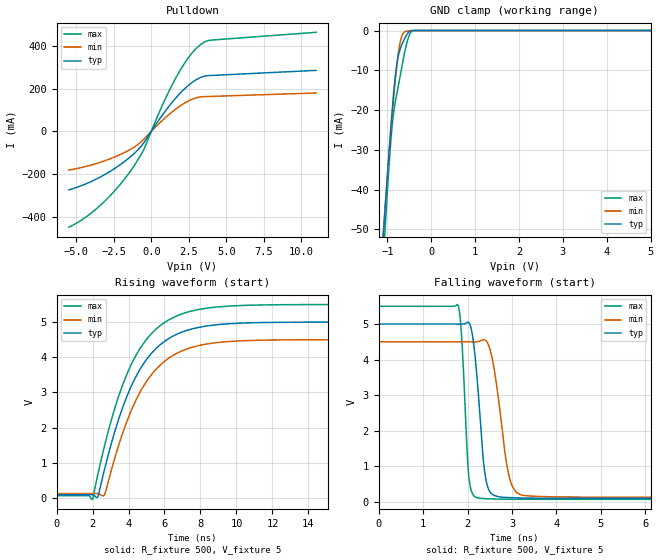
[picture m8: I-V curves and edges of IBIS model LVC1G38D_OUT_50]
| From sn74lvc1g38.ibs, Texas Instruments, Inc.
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[Model]   LVC1G38D_OUT_50
Model_type  Open_drain
Enable   Active-High
Vref =   5.0
Rref =   500
Cref =   50p
Vmeas =   2.5
| variable   typ   min   max
C_comp   3.59pF   2.67pF   5.07pF
| C_pulldown   6.34pF   4.47pF   9.75pF
| C_tri-state   3.59pF   2.67pF   5.07pF
[Temperature Range]   40   100   -40
| Ambient temperature   25   85   -40
[Voltage range]   5   4.5   5.5
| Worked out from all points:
|   slope of the pulldown table from 0 to 0.75 V, typ, clamps not added: 9.74 ohm
|   GND clamp passes 1 mA (typ) near -0.56 V on its own axis
|   rising waveform, R_fixture 500, V_fixture 5: 20-80 % time 2.33ns typ, 2.31ns min, 2.35ns max; typ from 0.091 V to 5 V
|   falling waveform, R_fixture 500, V_fixture 5: 20-80 % time 188ps typ, 277ps min, 125ps max; typ from 5 V to 0.091 V
[GND Clamp]
| LVC1G38D_OUT_50
|   Voltage   I(typ)   I(min)   I(max)
-5.5V     -916.4mA   -845.5mA   -1.045A
-1.09V    -50.76mA   -49.98mA   -56.67mA
-1.06V    -45.77mA   -45.39mA   -51.02mA
-1.045V   -43.3mA    -43.11mA   -48.24mA
-915mV    -23.14mA   -24.32mA   -26.62mA
-870mV    -17.04mA   -18.38mA   -21.54mA
-820mV    -11.32mA   -12.35mA   -17.86mA
-765mV    -7.029mA   -6.772mA   -14.61mA
-710mV    -4.653mA   -2.903mA   -11.41mA
-590mV    -1.618mA   -231.3uA   -4.549mA
-430mV    -5.996uA   -38.1uA    -30.86uA
5V        30.43pA    275.2pA    975.5pA
[Pulldown]
| LVC1G38D_OUT_50
|   Voltage   I(typ)   I(min)   I(max)
-5.5V     -273.4mA   -180.8mA   -448mA
-4.485V   -248.9mA   -166.3mA   -406.7mA
-3.435V   -214.6mA   -145.3mA   -347.9mA
-2.39V    -171.2mA   -118.1mA   -273.7mA
-1.44V    -121.8mA   -85.93mA   -190.7mA
-515mV    -55.2mA    -37.6mA    -87.68mA
715mV     73.64mA    49.68mA    118.1mA
1.685V    159.9mA    107mA      255.9mA
2.51V     217.1mA    143.2mA    347.6mA
3.26V     251.1mA    161mA      404.3mA
3.945V    261.2mA    163.3mA    426.7mA
11V       285.2mA    179.5mA    463.2mA
[Ramp]
| LVC1G38D_OUT_50
| variable   typ   min   max
dV/dt_r   2.99/2.33E-09   2.67/2.32E-09   3.33/2.35E-09
dV/dt_f   2.98/1.95E-10   2.66/2.90E-10   3.29/1.28E-10
R_load = 500
[Rising Waveform]
| LVC1G38D_OUT_50
R_fixture =   500
C_fixture =   0
L_fixture =   0
V_fixture =   5
V_fixture_min = 4.5
V_fixture_max = 5.5
|   Time   V(typ)   V(min)   V(max)
0s        91.33mV    120.7mV    62.82mV
2.01ns    91.31mV    120.7mV    -34.92mV
2.305ns   40.65mV    120.7mV    683.9mV
2.665ns   805.5mV    88.22mV    1.471V
3.365ns   2.097V     1.351V     2.755V
4.07ns    3.082V     2.382V     3.704V
5.245ns   4.093V     3.484V     4.655V
6.69ns    4.656V     4.113V     5.178V
10.38ns   4.973V     4.47V      5.474V
24.99ns   5V         4.5V       5.5V
[Falling Waveform]
| LVC1G38D_OUT_50
R_fixture =   500
C_fixture =   0
L_fixture =   0
V_fixture =   5
V_fixture_min = 4.5
V_fixture_max = 5.5
|   Time   V(typ)   V(min)   V(max)
0s        5V         4.5V       5.5V
1.785ns   4.999V     4.5V       5.527V
1.87ns    4.998V     4.5V       4.557V
2.03ns    5.039V     4.499V     683.9mV
2.255ns   2.83V      4.512V     97.86mV
2.365ns   1.041V     4.556V     84.43mV
2.48ns    324.5mV    4.379V     77.34mV
2.935ns   111.5mV    713.3mV    65.54mV
3.285ns   98.61mV    168.2mV    63.63mV
24.99ns   91.33mV    120.7mV    62.82mV
